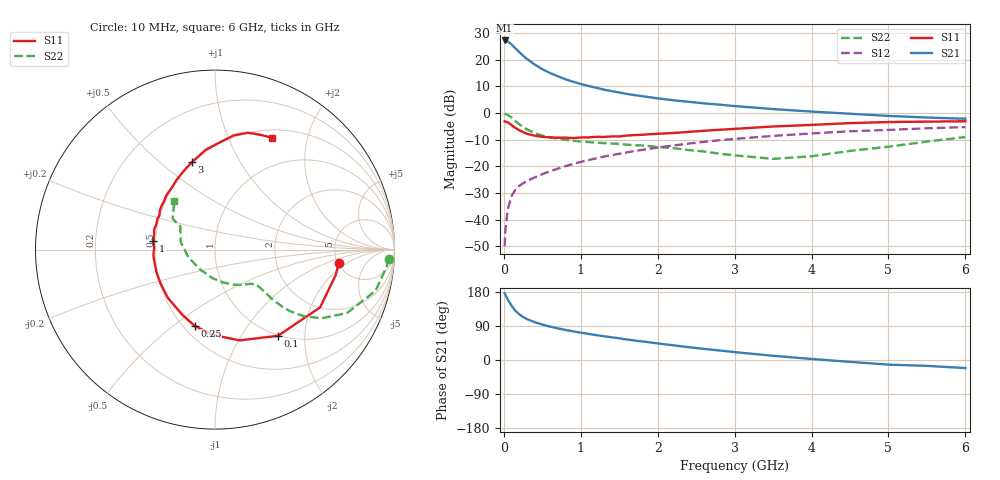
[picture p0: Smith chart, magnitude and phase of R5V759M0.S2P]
! SIEMENS Small Signal Semiconductors
! BFR183
! Si NPN RF Bipolar Junction Transistor in SOT23
! VCE = 0.75 V  IC = 9 mA
! Common Emitter S-Parameters:  May  1996
# GHz  S  MA  R  50
!  f  S11  S21  S12  S22
! GHz  MAG  ANG  MAG  ANG  MAG  ANG  MAG  ANG
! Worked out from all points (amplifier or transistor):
!   36 points, 10 MHz to 6 GHz, reference 50 ohm
!   highest |S21| = 27.2 dB at 10 MHz (marker M1)
!   |S21| within 3 dB of that: start of sweep to 152.5 MHz
!   unconditionally stable (mu >= 1): 709.1 MHz to 2.865 GHz
!   at 250 MHz: K = 0.61, MSG = 23.9 dB, |S12| = -26.3 dB
!   at 1.4 GHz: K = 1.08, MAG = 10.2 dB, |S12| = -15.8 dB
!   at 6 GHz: K = 0.95, MSG = 1.6 dB, |S12| = -5.3 dB
!   S11 on the Smith chart (normalised r, x): 10 MHz: 5.11, -1.45; 100 MHz: 0.99, -1.47; 250 MHz: 0.57, -0.60; 1 GHz: 0.49, +0.05; 3 GHz: 0.49, +0.64; 6 GHz: 0.60, +1.46
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0.01  0.694 -6.1  22.82 176.0  0.0032 86.8  0.9695 -3.0
0.02  0.6867 -12.1  22.64 171.6  0.0064 81.7  0.9603 -5.9
0.05  0.6683 -28.8  22.01 159.9  0.0154 76.2  0.9231 -14.4
0.1  0.5948 -53.8  19.27 143.4  0.0278 67.5  0.8154 -25.7
0.15  0.5243 -74.8  16.29 130.0  0.0365 61.8  0.7067 -32.8
0.2  0.4747 -91.8  13.88 120.6  0.043 58.6  0.6148 -37.0
0.25  0.4401 -104.9  11.82 113.6  0.0482 57.2  0.5438 -39.3
0.3  0.4074 -116.2  10.27 108.0  0.0532 57.3  0.4941 -40.3
0.4  0.376 -134.4  8.106 99.9  0.0621 57.4  0.4213 -40.9
0.5  0.3574 -147.9  6.605 93.3  0.0715 58.8  0.3752 -40.5
0.6  0.3498 -158.5  5.608 88.1  0.0809 59.7  0.3493 -40.3
0.7  0.3446 -167.0  4.877 83.5  0.0906 60.2  0.3299 -40.2
0.8  0.3451 -174.8  4.29 79.4  0.1008 60.4  0.3144 -40.3
1  0.3472 172.0  3.49 72.2  0.1209 60.8  0.2929 -41.0
1.1  0.3493 166.3  3.207 69.0  0.1309 60.5  0.2855 -42.3
1.6  0.3778 144.4  2.275 54.1  0.183 57.4  0.255 -49.2
2.2  0.4217 124.6  1.73 38.9  0.246 51.6  0.2198 -62.7
3  0.5035 104.8  1.348 20.8  0.3274 41.7  0.161 -94.1
3.5  0.5584 95.3  1.183 11.1  0.372 35.0  0.1382 -127.9
4.5  0.6455 80.6  0.968 -4.9  0.4547 21.8  0.1949 167.8
5.5  0.6883 68.2  0.822 -15.5  0.5173 10.1  0.2918 143.9
6  0.6994 63.0  0.779 -21.3  0.5448 2.6  0.3541 129.7
